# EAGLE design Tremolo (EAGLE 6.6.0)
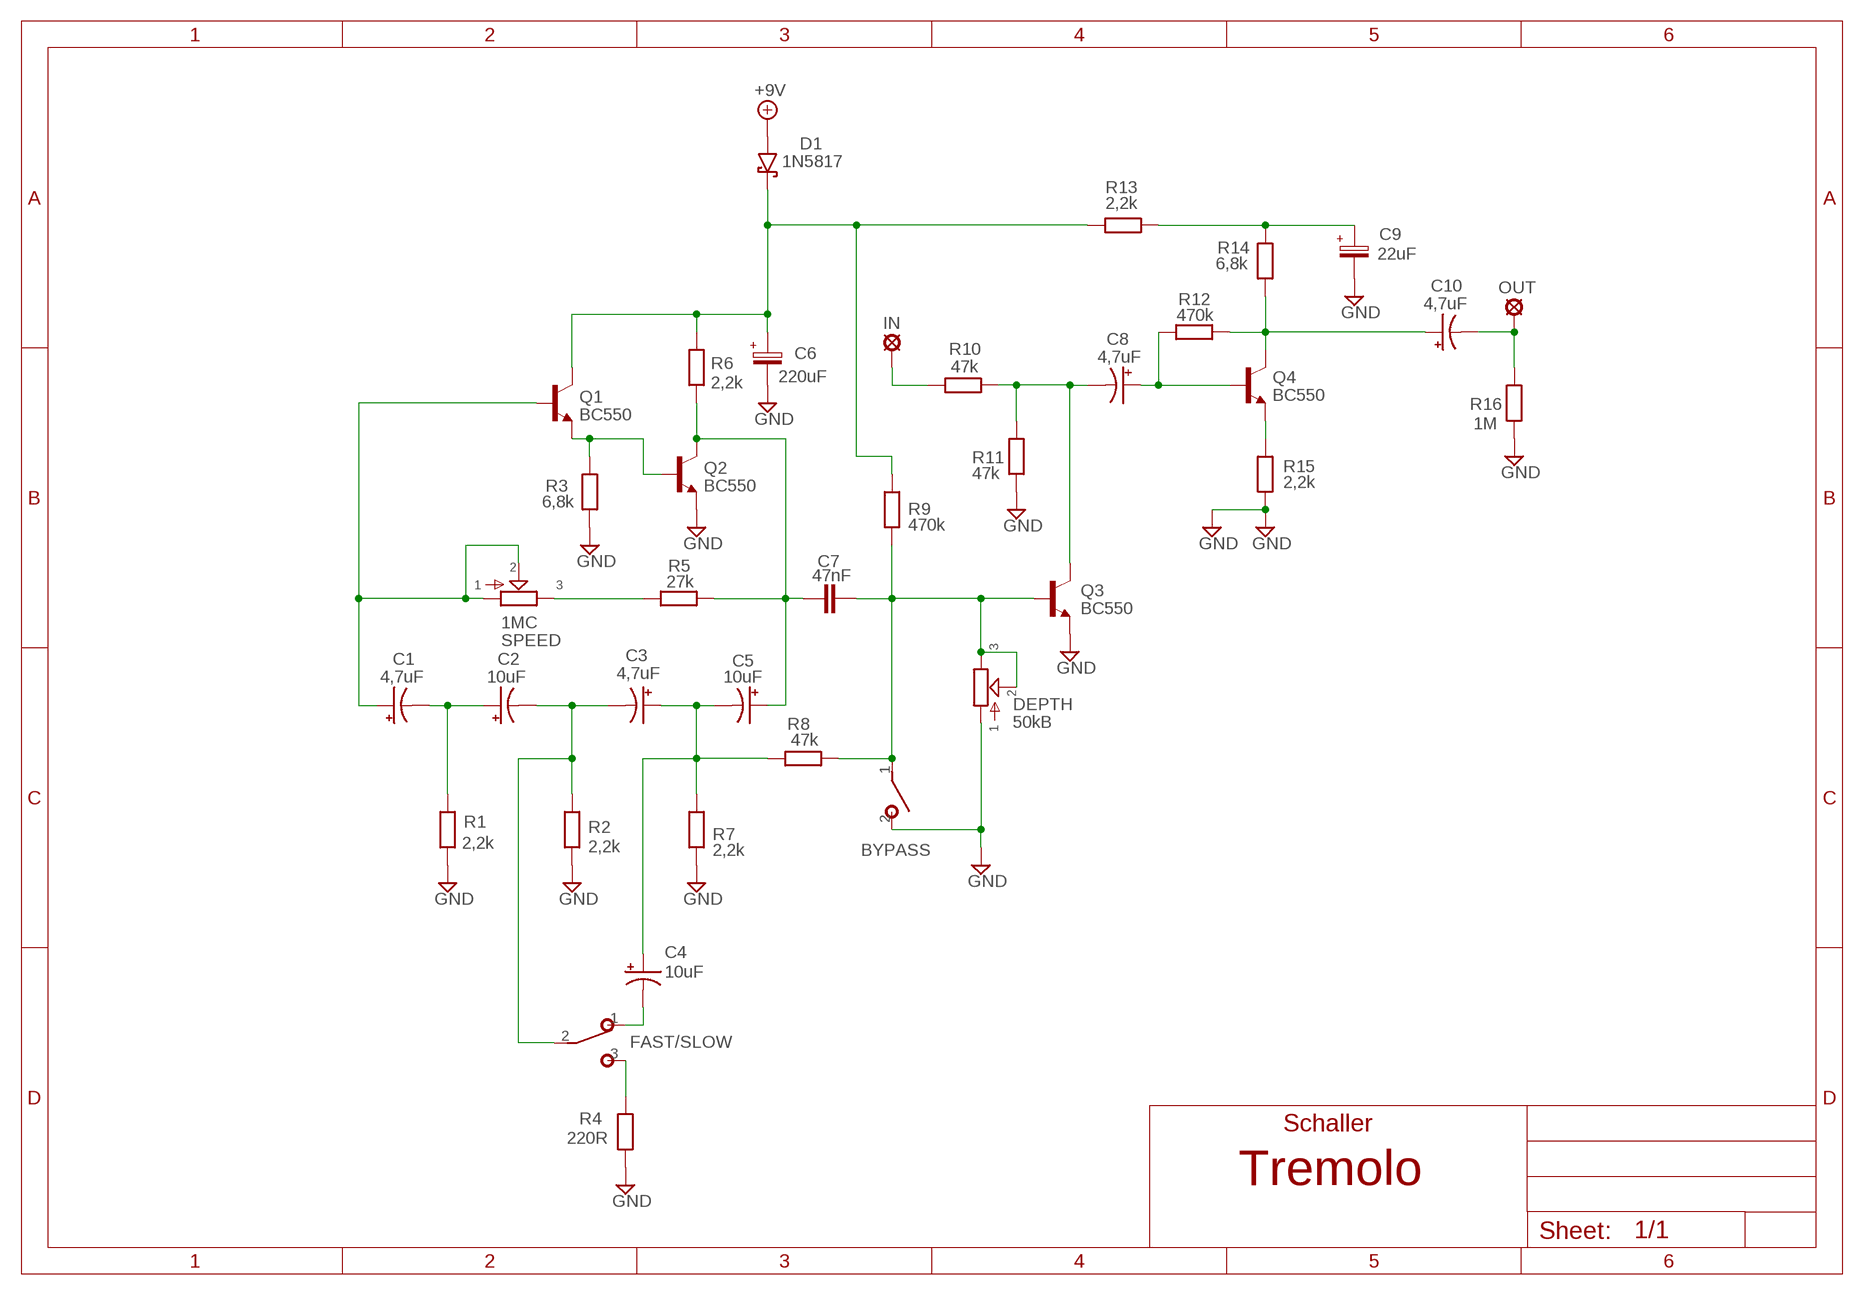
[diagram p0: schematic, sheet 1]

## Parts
+9V  +9V  +9V(T)1  [ROUND]
BYPASS  SPST  [SPST]
C1  4,7uF  044A1  [044A]
C2  10uF  044A1  [044A]
C3  4,7uF  044A1  [044A]
C4  10uF  044A1  [044A]
C5  10uF  044A1  [044A]
C6  220uF  063-EU  [063_025]
C7  47nF  22NF-82NF"  [4,5MM]
C8  4,7uF  044A1  [044A]
C9  22uF  063-EU  [063_025]
C10  4,7uF  044A1  [044A]
D1  1N5817  [DO41-3]
DEPTH  50kB  POT-EU16MM  [16MM]
FAST/SLOW  SPEED  SPDTPADS  [SPDT]
GND  GND  GND(T)1  [ROUND]
GND4  GND  GND(T)1  [ROUND]
IN  MCS10B  [MCS10B]
OUT  MCS10B  [MCS10B]
Q1  BC550  [TO92-]
Q2  BC550  [TO92-]
Q3  BC550  [TO92-]
Q4  BC550  [TO92-]
R1  2,2k  6MM-EU3  [R0207/3]
R2  2,2k  6MM-EU3  [R0207/3]
R3  6,8k  6MM-EU3  [R0207/3]
R4  220R  6MM-EU3  [R0207/3]
R5  27k  6MM-EU3  [R0207/3]
R6  2,2k  6MM-EU3  [R0207/3]
R7  2,2k  6MM-EU3  [R0207/3]
R8  47k  6MM-EU3  [R0207/3]
R9  470k  6MM-EU3  [R0207/3]
R10  47k  6MM-EU3  [R0207/3]
R11  47k  6MM-EU3  [R0207/3]
R12  470k  6MM-EU3  [R0207/3]
R13  2,2k  6MM-EU3  [R0207/3]
R14  6,8k  6MM-EU3  [R0207/3]
R15  2,2k  6MM-EU3  [R0207/3]
R16  1M  6MM-EU3  [R0207/3]
SPEED  1MC  POT-EU16MM  [16MM]

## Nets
+9V: +9V.1(+9V) D1.A
GND: BYPASS.2(S) C6.- C9.- DEPTH.1 GND4.1(GND) GND.1(GND) Q2.1(E) Q3.1(E) R1.1 R2.1 R3.1 R4.1 R7.1 R11.1 R15.2 R16.1
N$1: C9.+ R13.1 R14.2
N$2: C10.1(+) Q4.3(C) R12.1 R14.1
N$3: C8.1(+) Q4.2(B) R12.2
N$4: Q4.1(E) R15.1
N$5: C8.2(-) Q3.3(C) R10.2 R11.2
N$7: C6.+ D1.C Q1.3(C) R6.2 R9.2 R13.2
N$8: C10.2(-) OUT.MP R16.2
N$9: C1.1(+) Q1.2(B) SPEED.1 SPEED.2
N$12: C1.2(-) C2.1(+) R1.2
N$18: C2.2(-) C3.2(-) FAST/SLOW.2(P) R2.2
N$19: C3.1(+) C4.1(+) C5.2(-) R7.2 R8.2
N$20: R5.1 SPEED.3
N$21: Q1.1(E) Q2.2(B) R3.2
N$22: C5.1(+) C7.2 Q2.3(C) R5.2 R6.1
N$23: BYPASS.1(P) C7.1 DEPTH.2 DEPTH.3 Q3.2(B) R8.1 R9.1
N$24: C4.2(-) FAST/SLOW.1(O)
N$25: FAST/SLOW.3(S) R4.2
N$26: IN.MP R10.1

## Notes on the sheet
- Schaller

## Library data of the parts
+9V = gm-supply:+9V(T): +9V Voltage Supply
BYPASS = Kytkimet:SPST
C1-C5 C8 C10 = gm-caps-tant:044A: .1 - 1.5µF
C6 C9 = Elektrolyytit:063-EU
C7 = Mylar Kondensaattorit:22NF-82NF: 22nF-82nF
D1 = Diodit:1N5817
DEPTH SPEED = gm-pots:POT-EU
FAST/SLOW = Kytkimet:SPDT: TOGGLE SWITCH Marquardt
GND GND4 = gm-supply:GND(T): Ground
IN OUT = Padit:MCS10B: SOLDER PAD
Q1-Q4 = Transistorit:BC550
R1-R16 = Vastukset:6MM-EU: 6mm Resistors (European schematic symbol)

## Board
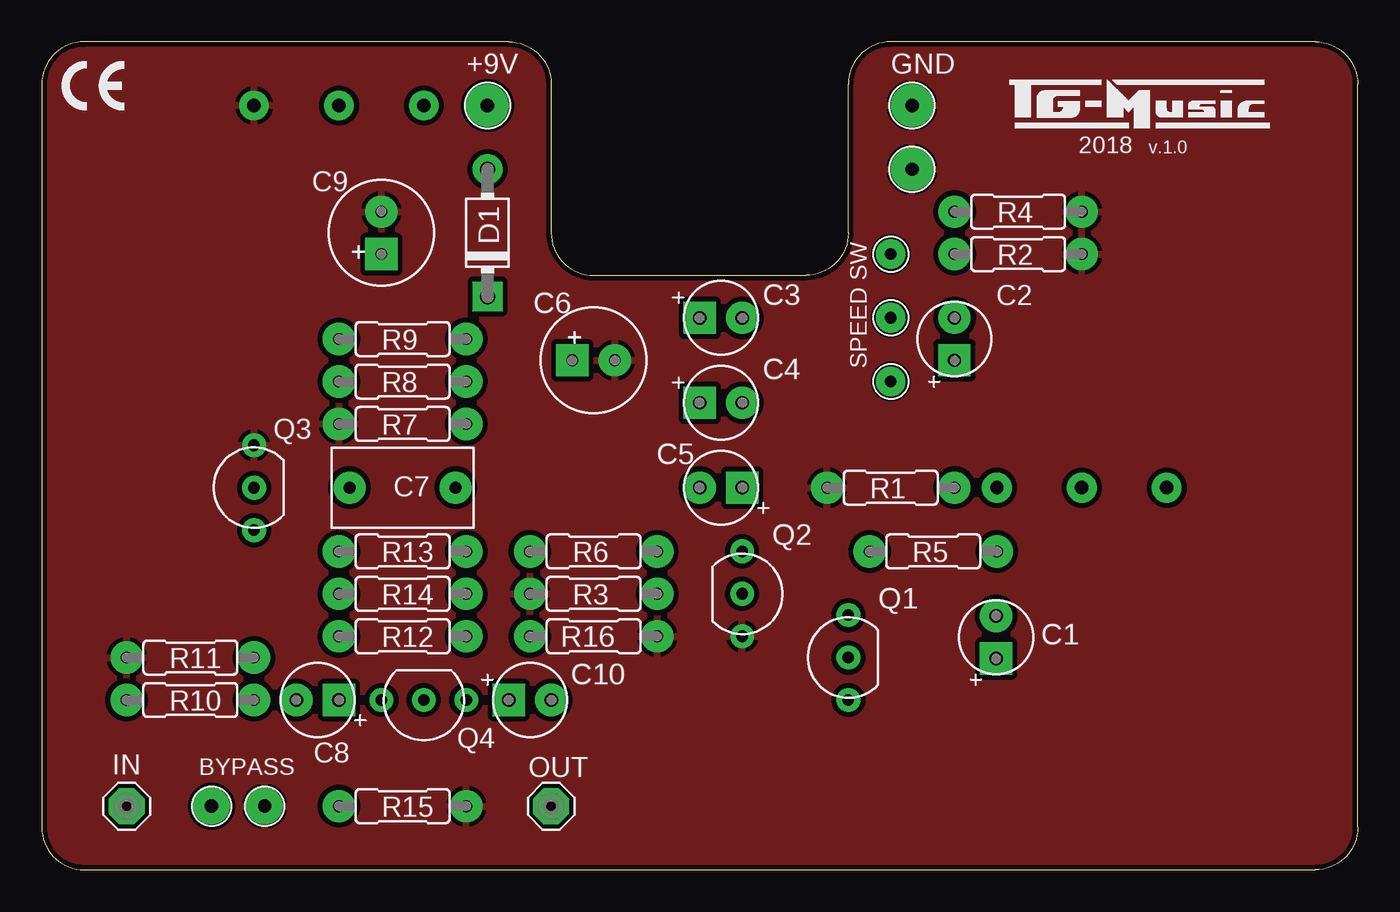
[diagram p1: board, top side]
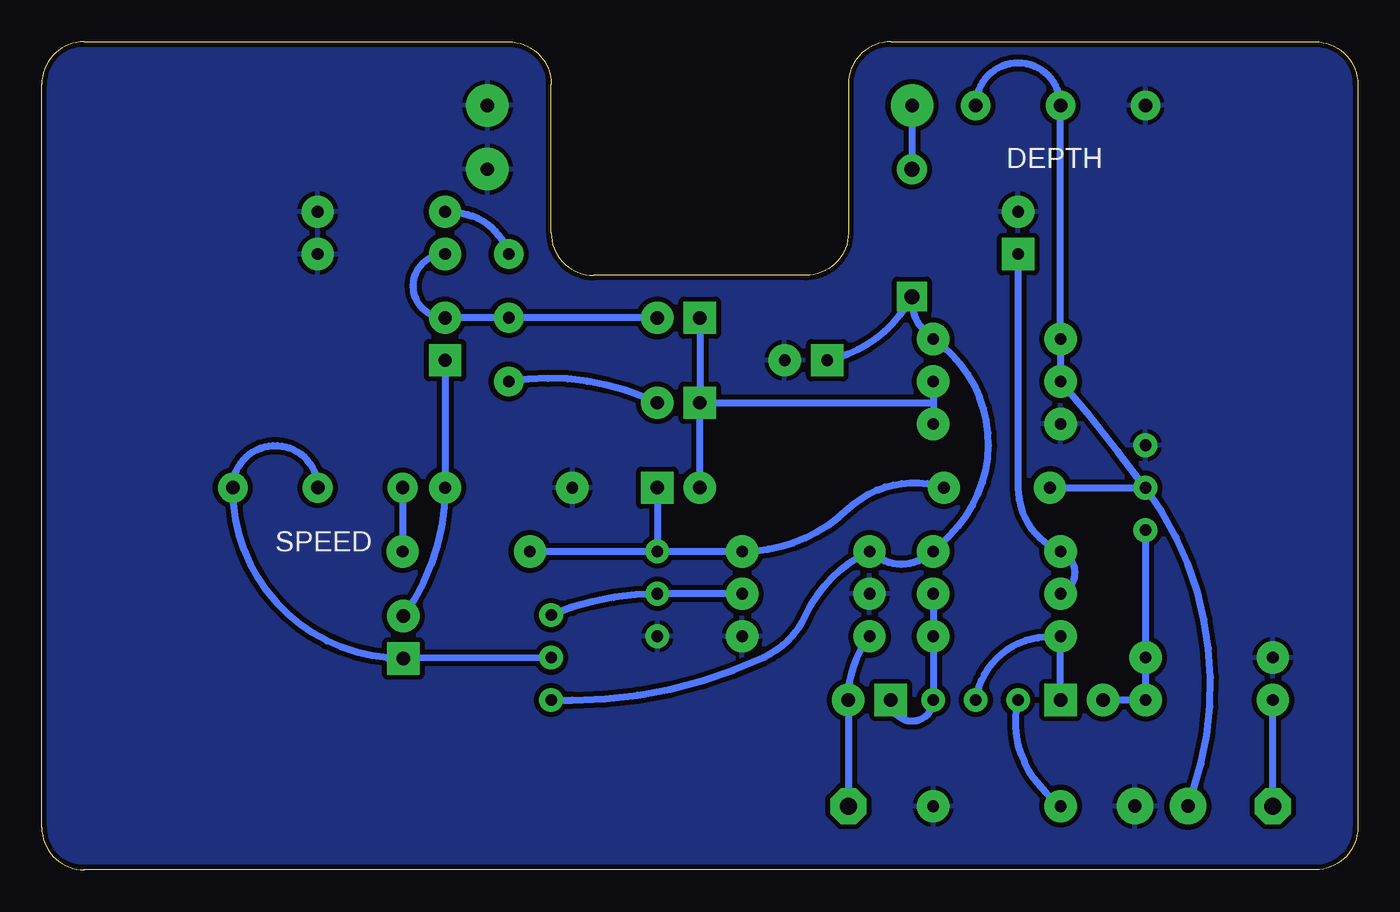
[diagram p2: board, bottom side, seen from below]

Size 78.74 x 49.53 mm. Coordinates in mm from the lower left corner, seen from the top.
Outline: 78.74,2.54 78.74,46.99 arc90 76.2,49.53 50.8,49.53 arc90 48.26,46.99 48.26,38.1 arc-90 45.72,35.56 33.02,35.56 arc-90 30.48,38.1 30.48,46.99 arc90 27.94,49.53 2.54,49.53 arc90 0,46.99 0,2.54 arc90 2.54,0 76.2,0 arc90 78.74,2.54
Copper layers (1*16): Top 0.035mm / dielectric 1.5mm / Bottom 0.035mm
Design rules "ITEADstudio": minimum track width 10mil, minimum drill 12mil, track to track 12mil, track to pad 12mil, pad to pad 12mil, via to via 12mil, smd to smd 0mil, copper to edge 12mil, drill to drill 12mil, minimum pad ring 10mil, minimum via ring 6mil, stop-mask expansion 4mil, vias tented up to drill 100mil, thermal gap 10mil

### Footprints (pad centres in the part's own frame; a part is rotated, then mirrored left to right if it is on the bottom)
ROUND = drill 0.8 pad 2.54: 1 0,0
SPST = drill 0.8 pad 2.184: 1 -1.27,0; 2 1.905,0
044A = drill 0.8 pad 1.93 square: 1 -1.27,0 | drill 0.8 pad 1.93: 2 1.27,0
063_025 = drill 0.7 pad 1.93 square: + -1.27,0 | drill 0.7 pad 1.93: - 1.27,0
4,5MM = drill 0.7 pad 1.93: 1 -3.175,0; 2 3.175,0
DO41-3 = drill 0.9 pad 1.778: A 3.81,0 | drill 0.9 pad 1.778 square: C -3.81,0
16MM = drill 0.8 pad 1.778: 1 5.08,0; 2 0,0; 3 -5.08,0
SPDT = drill 0.7 pad 1.778: 1 -3.81,0; 2 0,0; 3 3.81,0
MCS10B = drill 1.016 pad 2.159 octagon: MP 0,0
TO92- = drill 0.7 pad 1.422: 1 2.54,0; 2 0,0; 3 -2.54,0
R0207/3 = drill 0.7 pad 1.93: 1 -3.81,0; 2 3.81,0

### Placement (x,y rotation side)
+9V  26.67,45.72 0 top
BYPASS  11.43,3.81 0 top
C1  57.1,13.91 90 top
C2  54.61,31.75 90 top
C3  40.64,33.02 0 top
C4  40.64,27.94 0 top
C5  40.64,22.86 180 top
C6  33.02,30.48 0 top
C7  21.59,22.86 0 top
C8  16.51,10.16 180 top
C9  20.32,38.1 90 top
C10  29.21,10.16 0 top
D1  26.67,38.1 90 top
DEPTH  17.78,45.72 180 top
FAST/SLOW  50.8,33.02 90 top
GND  52.07,45.72 0 top
GND4  52.07,41.91 0 top
IN  5.08,3.81 0 top
OUT  30.48,3.81 0 top
Q1  48.26,12.7 90 top
Q2  41.91,16.51 270 top
Q3  12.7,22.86 90 top
Q4  22.86,10.16 180 top
R1  50.8,22.86 0 top
R2  58.42,36.83 180 top
R3  33.02,16.51 0 top
R4  58.42,39.37 180 top
R5  53.34,19.05 180 top
R6  33.02,19.05 180 top
R7  21.59,26.67 0 top
R8  21.59,29.21 0 top
R9  21.59,31.75 0 top
R10  8.89,10.16 0 top
R11  8.89,12.7 0 top
R12  21.59,13.97 180 top
R13  21.59,19.05 0 top
R14  21.59,16.51 180 top
R15  21.59,3.81 0 top
R16  33.02,13.97 180 top
SPEED  62.23,22.86 0 top

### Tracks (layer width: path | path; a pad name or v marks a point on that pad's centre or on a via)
+9V
  Bottom 0.406: +9V.1 D1.A
GND
  pour Bottom: 0,2.54 0,46.99 arc-90 2.54,49.53 27.94,49.53 arc-90 30.48,46.99 30.48,38.1 arc90 33.02,35.56 45.72,35.56 arc90 48.26,38.1 48.26,46.99 arc-90 50.8,49.53 76.2,49.53 arc-90 78.74,46.99 78.74,2.54 arc-90 76.2,0 2.54,0 arc-90
  pour Top: 0,2.54 0,46.99 arc-90 2.54,49.53 27.94,49.53 arc-90 30.48,46.99 30.48,38.1 arc90 33.02,35.56 45.72,35.56 arc90 48.26,38.1 48.26,46.99 arc-90 50.8,49.53 76.2,49.53 arc-90 78.74,46.99 78.74,2.54 arc-90 76.2,0 2.54,0 arc-90
N$1
  Bottom 0.406: C9.+ 20.32,22.86 arc-67 R13.1 arc135 R14.2
N$2
  Bottom 0.406: R14.1 R12.1 Q4.3 arc180 C10.1
N$3
  Bottom 0.406: Q4.2 arc78 18.73,13.92 R12.2 C8.1
N$4
  Bottom 0.406: R15.1 18.65,4.63 arc60 Q4.1
N$5
  Bottom 0.406: Q3.3 R11.2 R10.2 C8.2
N$7
  Bottom 0.406: C6.+ arc-46 27.04,33.71 D1.C arc-58 R9.2 arc101 24.4,20.02 R13.2 arc88 R6.2 arc-40 33.02,15.24 arc40 35.56,12.7 arc25 46.99,10.16 Q1.3
N$8
  Bottom 0.406: OUT.MP C10.2 arc37 R16.2
N$9
  Bottom 0.406: Q1.2 C1.1 arc91 SPEED.1 arc179 SPEED.2
N$12
  Bottom 0.406: C2.1 R1.2 arc36 C1.2
N$18
  Bottom 0.406: C3.2 FAST/SLOW.2 C2.2 arc180 R2.2
N$19
  Bottom 0.406: C3.1 C4.1 | C5.2 C4.1 | R8.2 25.4,27.94 | 25.4,27.94 R7.2 | C4.1 25.4,27.94
N$20
  Bottom 0.406: SPEED.3 R5.1
N$21
  Bottom 0.406: R3.2 Q2.2 arc-23 Q1.1
N$22
  Bottom 0.406: R5.2 Q2.3 | C5.1 Q2.3 | Q2.3 R6.1 arc-44 30.48,21.59 arc62 C7.2
N$23
  Bottom 0.406: BYPASS.1 9.87,4.67 arc-55 Q3.2 | DEPTH.3 arc180 DEPTH.2 R9.1 R8.1 arc4 Q3.2 | C7.1 Q3.2
N$24
  Bottom 0.406: C4.2 42.7,28.27 arc-32 FAST/SLOW.1
N$25
  Bottom 0.406: R4.2 53.88,39.31 arc68 FAST/SLOW.3
N$26
  Bottom 0.406: IN.MP R10.1

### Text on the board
tNames: 2018 | v.1.0 | SPEED SW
